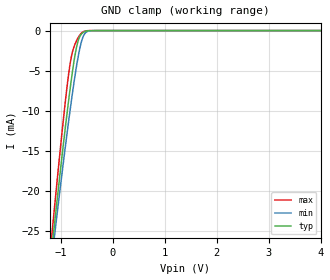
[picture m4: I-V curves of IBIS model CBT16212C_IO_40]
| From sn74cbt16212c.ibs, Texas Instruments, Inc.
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[Model]   CBT16212C_IO_40
Model_type  Terminator
| variable   typ   min   max
C_comp   8.32pF   6.56pF   12.64pF
| C_tri-state   8.32pF   6.56pF   12.64pF
[Temperature Range]   40   100   -40
| Ambient temperature   25   85   -40
[Voltage range]   4   4   4
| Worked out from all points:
|   GND clamp passes 1 mA (typ) near -0.65 V on its own axis
[GND Clamp]
| CBT16212C_IO_40
|   Voltage   I(typ)   I(min)   I(max)
-4V       -217.2mA   -203.1mA   -233.7mA
-1.165V   -26.95mA   -28.2mA    -25.19mA
-1.135V   -25.14mA   -26.53mA   -23.17mA
-1.105V   -23.33mA   -24.88mA   -21.17mA
-920mV    -12.64mA   -15mA      -9.438mA
-815mV    -7.1mA     -9.758mA   -4.012mA
-765mV    -4.747mA   -7.423mA   -2.466mA
-680mV    -1.666mA   -3.863mA   -1.075mA
-615mV    -555.1uA   -1.745mA   -419.6uA
-555mV    -182.6uA   -575uA     -116.6uA
-325mV    -1.226uA   -5.881uA   -41.54nA
4V        506.1pA    1.642nA    192.6pA
